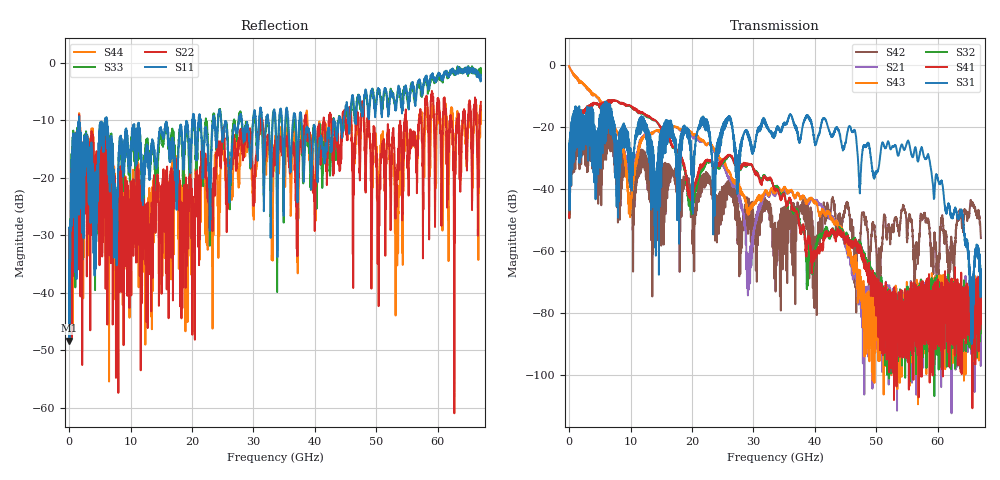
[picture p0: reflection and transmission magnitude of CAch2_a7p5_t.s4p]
!Agilent Technologies,N5247A,US51170199,A.09.90.13
!Agilent N5247A: A.09.90.13
!Date: Tuesday, October 23, 2018 14:30:05
!Correction: S11(Full 4 Port(1,2,3,4))
!S12(Full 4 Port(1,2,3,4))
!S13(Full 4 Port(1,2,3,4))
!S14(Full 4 Port(1,2,3,4))
!S21(Full 4 Port(1,2,3,4))
!S22(Full 4 Port(1,2,3,4))
!S23(Full 4 Port(1,2,3,4))
!S24(Full 4 Port(1,2,3,4))
!S31(Full 4 Port(1,2,3,4))
!S32(Full 4 Port(1,2,3,4))
!S33(Full 4 Port(1,2,3,4))
!S34(Full 4 Port(1,2,3,4))
!S41(Full 4 Port(1,2,3,4))
!S42(Full 4 Port(1,2,3,4))
!S43(Full 4 Port(1,2,3,4))
!S44(Full 4 Port(1,2,3,4))
!S4P File: Measurements: <S11,S12,S13,S14>,
!<S21,S22,S23,S24>,
!<S31,S32,S33,S34>,
!<S41,S42,S43,S44>:
# Hz S  dB  R 50
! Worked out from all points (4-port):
!   6701 points, 10 MHz to 67 GHz, reference 50 ohm
!   strongest paths, dB at 10 MHz, 16.76 GHz, 33.51 GHz, 50.25 GHz, 67 GHz:
!     S31: -33.3, -23.1, -21.6, -33.9, -70.4
!     S41: -48.5, -25.7, -40.2, -75.6, -73.6
!     S32: -48.4, -25.9, -39.6, -70.4, -86.5
!     S43: -0.3, -20.0, -41.0, -85.2, -78.7
!     S21: -0.4, -19.9, -41.8, -72.5, -76.5
!     S42: -33.5, -35.1, -50.8, -73.1, -55.8
!   lowest |S11| = -48.3 dB at 59.99 MHz (marker M1), VSWR 1.01, Z = 50.4 + j0.0433 ohm
!   |S11| at or under -10 dB: 1.644 GHz to 5.888 GHz (4.244 GHz wide, 113 % of centre); 6.191 GHz to 20.06 GHz (13.86 GHz wide, 106 % of centre); 37.84 GHz to 43.09 GHz (5.249 GHz wide, 13 % of centre)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
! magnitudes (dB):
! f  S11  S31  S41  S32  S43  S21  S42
! 10 MHz  -28.7  -33.3  -48.5  -48.4  -0.3  -0.4  -33.5
! 59.99 MHz  -48.3  -28.0  -47.8  -47.9  -0.7  -0.7  -28.5
! 7.669 GHz  -27.1  -25.4  -11.5  -11.5  -20.9  -21.1  -29.9
! 9.929 GHz  -17.3  -33.2  -13.0  -13.2  -49.0  -38.1  -35.4
! 19.59 GHz  -15.5  -23.5  -42.1  -45.1  -21.3  -21.9  -38.8
! 55.13 GHz  -6.9  -24.4  -76.8  -80.8  -78.6  -78.2  -52.3
! 67 GHz  -2.1  -70.4  -73.6  -86.5  -78.7  -76.5  -55.8
